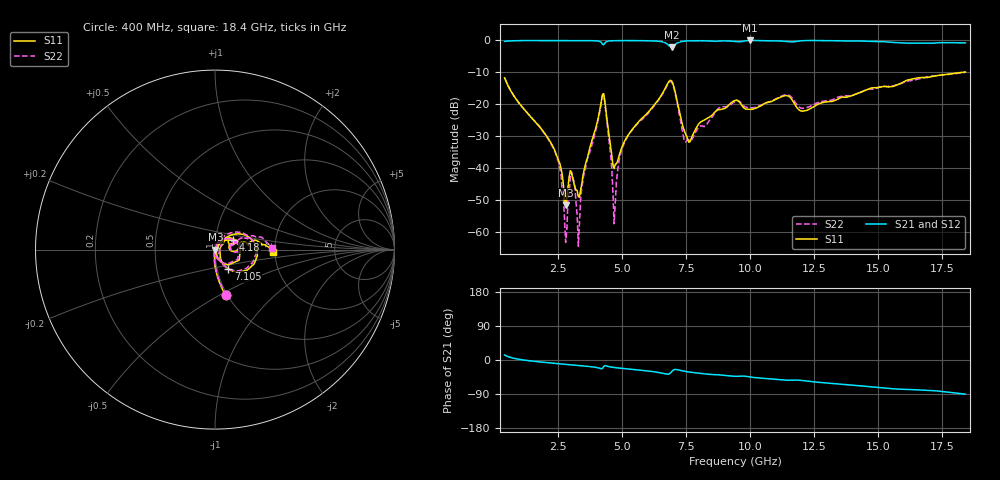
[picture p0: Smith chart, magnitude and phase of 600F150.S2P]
!  American Technical Ceramics  Date:  12/6/06
!  One Norden Lane
!  Huntington Station,  NY.  11746-2102
!  Tel:  (631) 622-4700  Fax:  (631) 622-4748
!  Part Number  600F150  Mounting Orientation: Horizontal
!  Description: Ultra Low ESR Microwave capacitors
!  Application: Coupling, Bypass, Tuning, DC Block
!  Filters, Matching
# GHZ S DB R 50
! Freq  |S11|  S11 Ph  |S21|  S21 Ph  |S12|  S12 Ph  |S22|  S22 Ph
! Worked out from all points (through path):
!   401 points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, 400 MHz to 18.4 GHz, reference 50 ohm
!   highest |S21| = 0.00 dB at 9.985 GHz (marker M1); lowest = -2.2 dB at 6.925 GHz (marker M2)
!   group delay of S21, straight-line fit = 14 ps
!   lowest |S11| = -51.6 dB at 2.785 GHz (marker M3), VSWR 1.01, Z = 50.3 - j0.0833 ohm
!   |S11| at or under -10 dB: start of sweep to 18.24 GHz
!   |S22| runs from -64.3 to -10.0 dB; largest |S21 - S12| = 0.0015
!   S11 on the Smith chart (normalised r, x): 400 MHz: 0.98, -0.53; 4.18 GHz: 1.22, +0.13; 7.105 GHz: 1.13, -0.25; 18.4 GHz: 1.94, -0.06
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0.4  -11.69 -76.9  -0.31 13.3  -0.31 13.3  -11.66 -76.0
2.29  -33.19 -91.6  -0.02 -8.4  -0.02 -8.4  -33.40 -103.3
2.515  -37.64 -85.4  -0.02 -9.8  -0.02 -9.8  -38.27 -111.2
2.785  -51.56 -18.3  -0.03 -11.5  -0.03 -11.5  -63.14 160.2
3.01  -41.37 -83.6  -0.04 -12.8  -0.04 -12.8  -40.93 -95.5
3.28  -48.90 -22.0  -0.04 -14.3  -0.04 -14.3  -64.32 15.1
3.415  -44.84 38.5  -0.03 -15.2  -0.03 -15.2  -45.93 73.1
4.18  -18.84 28.4  -0.66 -23.1  -0.66 -23.1  -19.30 33.3
4.36  -22.09 -63.8  -0.47 -15.3  -0.47 -15.3  -22.90 -67.7
4.63  -38.84 -46.8  -0.08 -19.2  -0.08 -19.2  -47.16 -90.5
4.72  -38.73 -3.5  -0.04 -20.1  -0.04 -20.1  -51.35 48.9
5.08  -31.57 46.3  -0.04 -22.8  -0.04 -22.8  -31.90 72.7
6.43  -18.27 41.8  -0.26 -33.2  -0.26 -33.2  -18.53 49.2
6.925  -12.68 -20.1  -2.18 -30.8  -2.18 -30.8  -13.04 -18.3
7.105  -17.67 -55.8  -0.99 -25.0  -0.99 -25.1  -18.24 -56.7
7.6  -31.84 -8.9  -0.14 -31.8  -0.14 -31.8  -31.11 -2.4
9.4  -18.78 30.7  -0.30 -43.1  -0.31 -43.1  -19.00 29.6
9.985  -21.55 26.4  0.00 -44.7  0.00 -44.8  -21.04 19.2
11.38  -17.25 13.2  -0.32 -53.4  -0.31 -53.4  -17.01 9.7
12.415  -20.98 19.6  -0.01 -57.2  -0.01 -57.2  -20.28 17.9
15.43  -14.52 8.2  -0.53 -75.3  -0.53 -75.3  -14.35 18.4
18.4  -9.88 -2.3  -0.77 -90.1  -0.76 -90.1  -9.96 1.6
